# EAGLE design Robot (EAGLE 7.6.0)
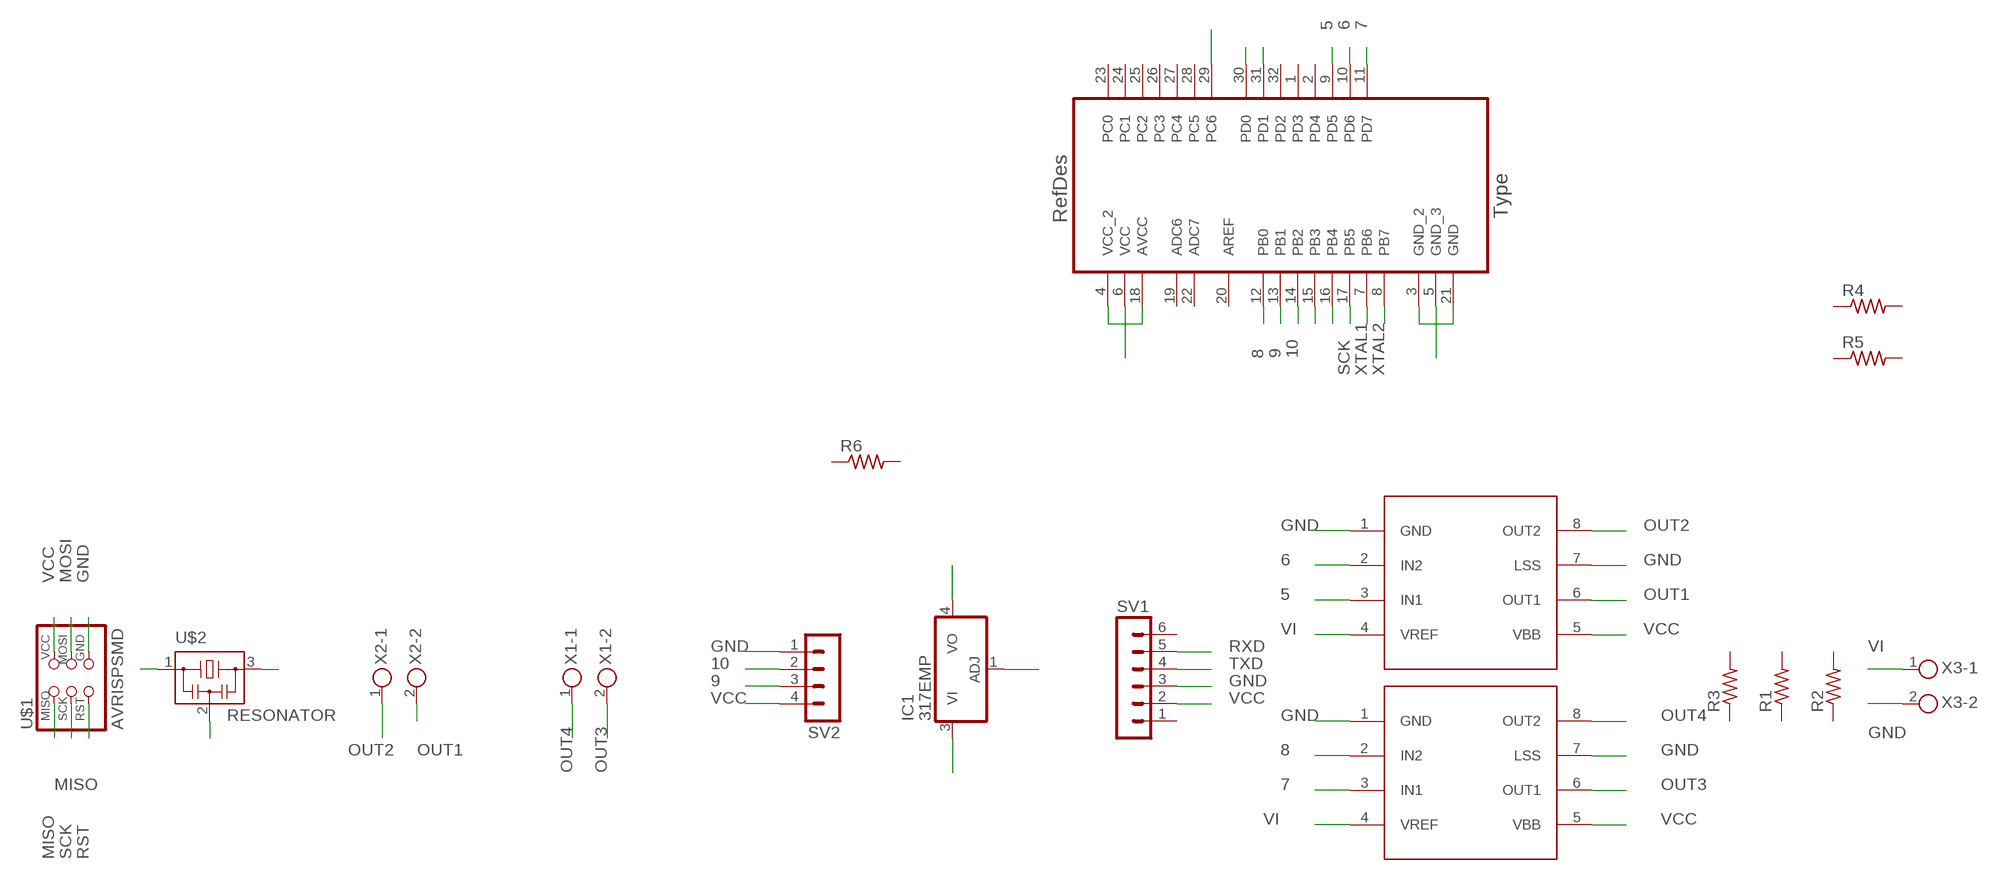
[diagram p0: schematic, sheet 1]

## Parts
IC1  317EMP  [SOT223]
R1  RES-US1206FAB  [R1206FAB]
R2  RES-US1206FAB  [R1206FAB]
R3  RES-US1206FAB  [R1206FAB]
R4  RES-US1206FAB  [R1206FAB]
R5  RES-US1206FAB  [R1206FAB]
R6  RES-US1206FAB  [R1206FAB]
SV1  MA06-1  [MA06-1]
SV2  MA04-1  [MA04-1]
U1  ATMEGA328P-AU  [QFP80P900X900X120-32N]
U$1  AVRISPSMD  [2X03SMD]
U$2  RESONATOR  [EFOBM]
U$3  A4953-H-BRIDGE-MOTOR-DRIVER  [SOIC8]
U$4  A4953-H-BRIDGE-MOTOR-DRIVER  [SOIC8]
X1  AKL59-02  [2POL35]
X2  AKL59-02  [2POL35]
X3  AKL59-02  [2POL35]

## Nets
5: U1.9(PD5) U$3.3(IN1)
6: U1.10(PD6) U$3.2(IN2)
7: U1.11(PD7) U$4.3(IN1)
8: U1.12(PB0) U$4.2(IN2)
9: SV2.3 U1.13(PB1)
10: SV2.2 U1.14(PB2)
GND: IC1.4(VO) SV1.3 SV2.1 U1.3(GND_2) U1.5(GND_3) U1.21(GND) U$1.6(GND) U$2.2 U$3.1(GND) U$3.7(LSS) U$4.1(GND) U$4.7(LSS) X3.2
MISO: U1.16(PB4) U$1.1(MISO)
MOSI: U1.15(PB3) U$1.4(MOSI)
OUT1: U$3.6(OUT1) X2.2
OUT2: U$3.8(OUT2) X2.1
OUT3: U$4.6(OUT1) X1.2
OUT4: U$4.8(OUT2) X1.1
RST: U1.29(PC6) U$1.5(RST)
RXD: SV1.5 U1.31(PD1)
SCK: U1.17(PB5) U$1.3(SCK)
TXD: SV1.4 U1.30(PD0)
VCC: IC1.3(VI) SV1.2 SV2.4 U1.4(VCC_2) U1.6(VCC) U1.18(AVCC) U$1.2(VCC) U$3.5(VBB) U$4.5(VBB)
VI: IC1.1(ADJ) U$3.4(VREF) U$4.4(VREF) X3.1
XTAL1: U1.7(PB6) U$2.3
XTAL2: U1.8(PB7) U$2.1
Unconnected: R1.1 R1.2 R2.1 R2.2 R3.1 R3.2 R4.1 R4.2 R5.1 R5.2 R6.1 R6.2 SV1.1 SV1.6 U1.1(PD3) U1.2(PD4) U1.19(ADC6) U1.20(AREF) U1.22(ADC7) U1.23(PC0) U1.24(PC1) U1.25(PC2) U1.26(PC3) U1.27(PC4) U1.28(PC5) U1.32(PD2)

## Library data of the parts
IC1 = linear:*317: Positive VOLTAGE REGULATOR
R1-R6 = fab:RES-US: Resistor (US Symbol)
SV1 = con-lstb:MA06-1: PIN HEADER; OC_FARNELL: unknown; OC_NEWARK: unknown
SV2 = con-lstb:MA04-1: PIN HEADER; OC_FARNELL: unknown; OC_NEWARK: unknown
U1 = Atmel-ATMEGA328P-AU:ATMEGA328P-AU; DESCRIPTION: 8-bit Microcontroller with In-System Programmable Flash; MPN: ATMEGA328P-AU; OC_FARNELL: 1715486; OC_NEWARK: 14R4631; PACKAGE: TQFP-32; SUPPLIER: Atmel
U$1 = fab:AVRISP
U$2 = fab:RESONATOR
U$3 U$4 = fab:A4953-H-BRIDGE-MOTOR-DRIVER
X1-X3 = con-ria-59:AKL59-02: RIA Anschlussklemme Typ 59, Raster 3,5 mm, Polzahl 2

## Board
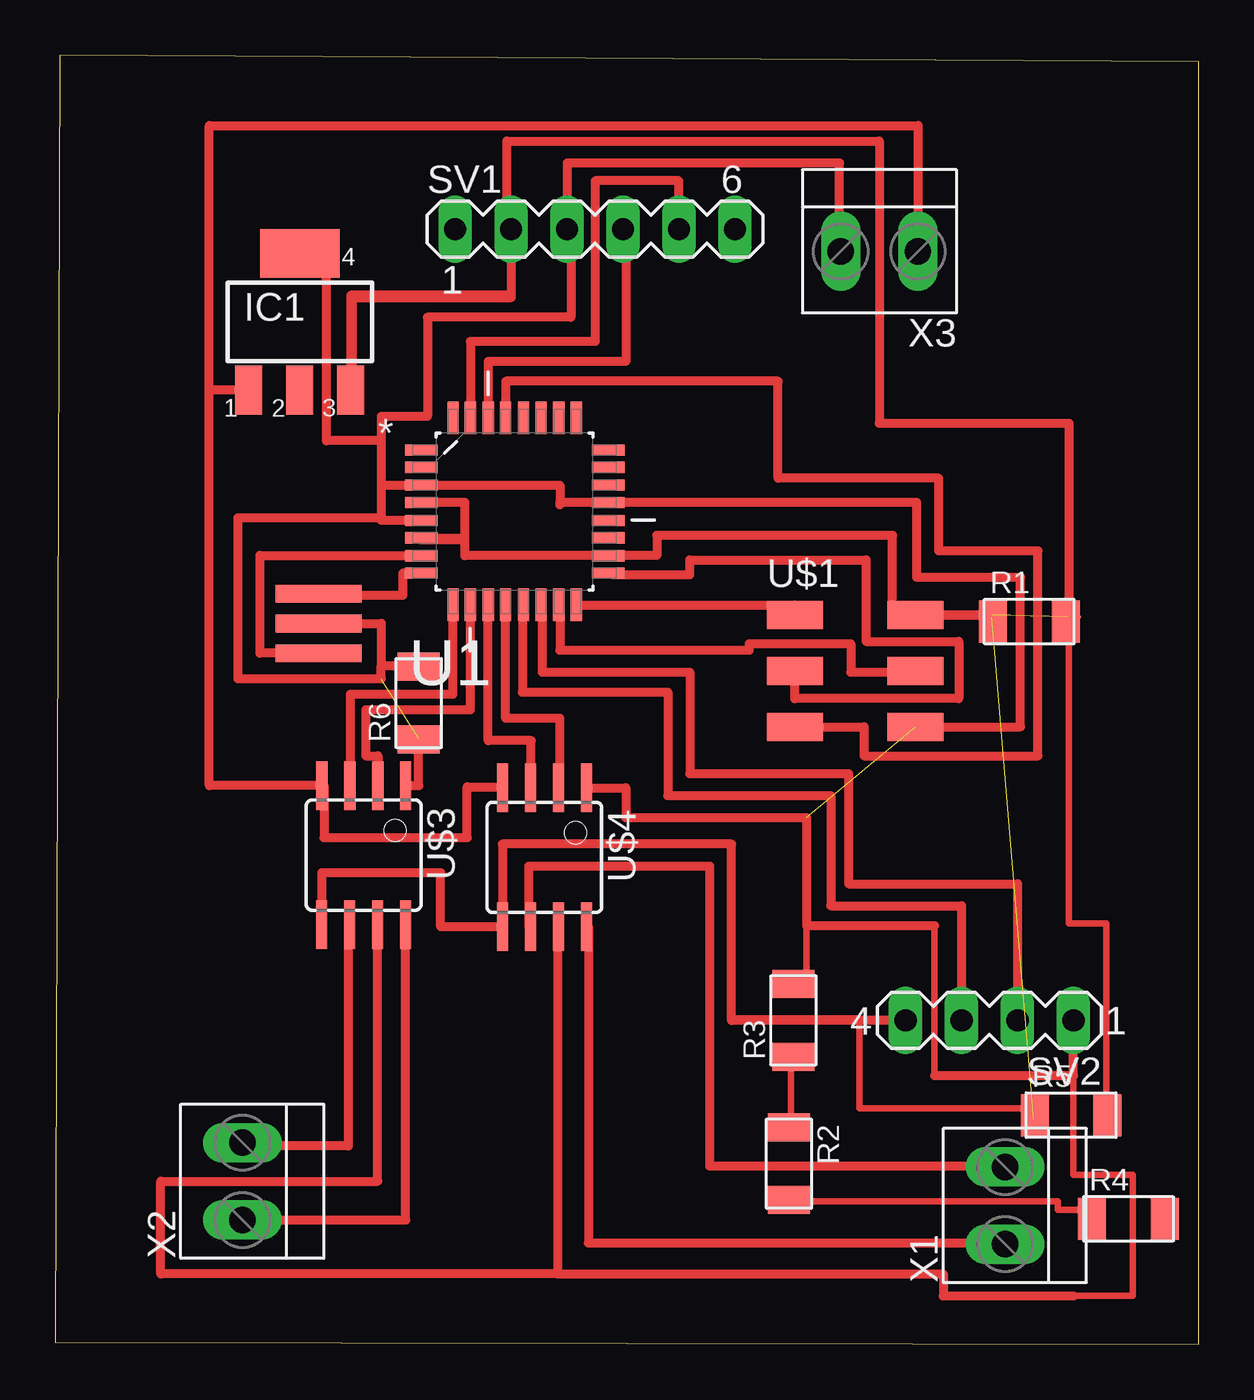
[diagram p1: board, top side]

Size 51.9 x 58.5 mm. Coordinates in mm from the lower left corner, seen from the top.
Outline: 0,0.1 51.9,0 51.9,58.2 0.2,58.5 0,0.1
Copper layers (1*16): Top 0.035mm / dielectric 1.5mm / Bottom 0.035mm
Design rules "default": minimum track width 10mil, minimum drill 24mil, track to track 8mil, track to pad 8mil, pad to pad 8mil, via to via 8mil, smd to smd 8mil, copper to edge 40mil, drill to drill 8mil, minimum pad ring 10mil, minimum via ring 8mil, stop-mask expansion 4mil, vias tented up to drill 0mil, thermal gap 10mil

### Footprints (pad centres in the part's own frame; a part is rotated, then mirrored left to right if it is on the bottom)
SOT223 = smd 1.219 x 2.235: 1 -2.311,-3.099; 2 0,-3.099; 3 2.311,-3.099 | smd 3.6 x 2.2: 4 0,3.099
R1206FAB = smd 1.27 x 1.905: 1 -1.651,0; 2 1.651,0
MA06-1 = drill 1.016 long: 1 -6.35,0; 2 -3.81,0; 3 -1.27,0; 4 1.27,0; 5 3.81,0; 6 6.35,0
MA04-1 = drill 1.016 long: 1 -3.81,0; 2 -1.27,0; 3 1.27,0; 4 3.81,0
QFP80P900X900X120-32N = smd 1.473 x 0.508: 1 -4.242,2.794; 2 -4.242,2.007; 3 -4.242,1.194; 4 -4.242,0.406; 5 -4.242,-0.406; 6 -4.242,-1.194; 7 -4.242,-2.007; 8 -4.242,-2.794; 17 4.242,-2.794; 18 4.242,-2.007; 19 4.242,-1.194; 20 4.242,-0.406; 21 4.242,0.406; 22 4.242,1.194; 23 4.242,2.007; 24 4.242,2.794 | smd 0.508 x 1.473: 9 -2.794,-4.242; 10 -2.007,-4.242; 11 -1.194,-4.242; 12 -0.406,-4.242; 13 0.406,-4.242; 14 1.194,-4.242; 15 2.007,-4.242; 16 2.794,-4.242; 25 2.794,4.242; 26 2.007,4.242; 27 1.194,4.242; 28 0.406,4.242; 29 -0.406,4.242; 30 -1.194,4.242; 31 -2.007,4.242; 32 -2.794,4.242
2X03SMD = smd 2.54 x 1.27: 1 -2.54,2.54; 2 2.92,2.54; 3 -2.54,0; 4 2.92,0; 5 -2.54,-2.54; 6 2.92,-2.54
EFOBM = smd 0.8 x 3.9: 1 -1.35,0; 2 0,0; 3 1.35,0
SOIC8 = smd 0.5 x 2.2: 1 -1.905,-3.154; 2 -0.645,-3.154; 3 0.625,-3.154; 4 1.895,-3.154; 5 1.905,3.154; 6 0.635,3.154; 7 -0.635,3.154; 8 -1.905,3.154
2POL35 = drill 1.2 long: 1 -1.75,0; 2 1.75,0

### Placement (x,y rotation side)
IC1  11.1,46.4 0 top
R1  44.2,32.8 0 top
R2  33.3,8.2 270 top
R3  33.5,14.7 90 top
R4  48.7,5.7 0 top
R5  46.1,10.4 0 top
R6  16.5,29.1 90 top
SV1  24.5,50.6 0 top
SV2  42.4,14.7 180 top
U1  20.85,37.79 0 top
U$1  36.11,30.56 0 top
U$2  11.96,32.71 270 top
U$3  14,22.2 180 top
U$4  22.2,22.1 180 top
X1  43.1,6.3 90 top
X2  8.5,7.4 90 top
X3  37.4,49.6 180 top

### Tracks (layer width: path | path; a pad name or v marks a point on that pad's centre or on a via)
5
  Top 0.406: U$3.3 13.4,25.35 13.4,29.5 18.06,29.5 U1.9
6
  Top 0.406: 14.7,25.35 U$3.2 14.65,26.7 14.1,26.7 14.1,28.8 18.84,28.8 U1.10
7
  Top 0.406: U$4.3 21.6,25.25 21.6,27.4 19.66,27.4 U1.11
8
  Top 0.406: U$4.2 22.9,25.25 22.9,28.4 20.44,28.4 U1.12
9
  Top 0.406: U1.13 21.2,33.55 21.2,29.6 27.8,29.6 27.8,24.9 35.2,24.9 35.2,19.9 41.13,19.9 SV2.3
10
  Top 0.406: U1.14 22.1,33.55 22.1,30.5 28.8,30.5 28.8,25.9 36,25.9 36,20.9 43.67,20.9 SV2.2
GND  (2 unrouted)
  Top 0.305: 39.9,19 39.9,12.2 | 46.21,2.2 48.9,2.2 48.9,7.7 46.21,7.7 46.21,12.2 | 33.4,16.3 34.1,16.3 34.1,19
  Top 0.406: 22.9,38.2 22.9,38.98 U1.3 16.61,39 14.8,39 | 22.9,38.2 U1.21 39.1,38.2 39.1,34.8 43.8,34.8 43.8,28.02 U$1.6 | 22.9,38.2 22.9,38.1 | X3.2 35.6,49.6 35.6,53.6 23.23,53.6 SV1.3 23.4,50.6 23.4,46.6 16.9,46.6 16.9,42.1 14.8,42.1 14.8,41 | U1.5 14.8,37.38 14.8,37.5 | U$2.2 14.8,32.71 14.8,30.8 | 14.8,39 14.8,37.5 | 14.8,37.5 8.3,37.5 8.3,30.2 14.8,30.2 14.8,30.8 | 14.8,41 14.8,39 | 22.8,3.2 4.8,3.2 4.8,7.4 14.63,7.4 U$3.7 | U$4.1 25.9,25.25 25.9,23.9 34.1,23.9 34.1,19 39.9,19 | 39.9,12.2 46.21,12.2 SV2.1 | U$4.7 22.8,18.95 22.8,3.2 | 22.8,3.2 40.3,3.2 40.3,2.2 46.21,2.2 | IC1.4 12.3,49.5 12.3,41 14.8,41 | 14.8,30.8 16.6,30.8 | U$3.1 16.5,25.35 16.5,27.5
MISO
  Top 0.406: U1.16 33.57,33.55 U$1.1
MOSI
  Top 0.406: U1.15 22.9,33.55 22.9,31.5 31.5,31.5 31.5,31.8 36.1,31.8 36.1,30.5 39.03,30.5 U$1.4
N$1
  Top 0.406: 42.7,33.1 39.1,33.1 39.1,33.3
N$2
  Top 0.305: 46.4,33 46,33 46,19.1 47.7,19.1 47.7,10.3
N$3
  Top 0.305: 47,6.1 45.5,6.1 45.5,6.5 33.3,6.5
N$4
  Top 0.406: 10.9,49.3 10.9,49.4
N$5
  Top 0.305: 33.1,9.8 33.4,9.8 33.4,13.3
OUT1
  Top 0.406: U$3.6 13.3,19.05 13.3,9 8.5,9 X2.2
OUT2
  Top 0.406: X2.1 15.91,5.65 U$3.8
OUT3
  Top 0.406: U$4.6 21.5,18.95 21.5,21.7 29.7,21.7 29.7,8.1 43.1,8.1 X1.2
OUT4
  Top 0.406: U$4.8 24.2,18.95 24.2,4.6 43.1,4.6 X1.1
RST
  Top 0.406: U$1.5 36.7,28.02 36.7,26.7 44.6,26.7 44.6,36 40.1,36 40.1,39.3 32.8,39.3 32.8,43.7 20.44,43.7 U1.29
RXD
  Top 0.406: SV1.5 28.3,49.5 28.3,52.8 24.5,52.8 24.5,45.5 18.84,45.5 U1.31
SCK
  Top 0.254: 25.3,34.92 U1.17
  Top 0.406: 25.3,34.92 28.8,34.92 28.8,35.6 36.8,35.6 36.8,31.9 41,31.9 41,29.3 33.57,29.3 U$1.3
TXD
  Top 0.406: SV1.4 25.9,49.5 25.9,44.6 19.66,44.6 U1.30
VCC  (2 unrouted)
  Top 0.305: 30.7,14.8 36.5,14.8 36.5,10.7 44.4,10.7 44.4,10.2
  Top 0.406: U1.4 18.6,38.2 18.6,36.6 U1.6 16.61,36.5 18.6,36.5 18.6,35.78 U1.18 25.09,35.8 27.3,35.8 27.3,36.7 38,36.7 38,33.1 U$1.2 42.5,33.1 42.5,33 | U$3.5 12.09,21.4 17.5,21.4 17.5,18.95 U$4.5 20.3,22.7 30.7,22.7 30.7,14.8 30.7,14.7 SV2.4 | SV1.2 20.7,50.5 | 20.7,50.5 20.7,47.6 | 20.7,47.6 13.41,47.6 IC1.3 13.5,43.3 13.5,47.5 20.7,47.5 20.7,47.6 | 20.7,50.5 20.5,50.5 20.5,54.6 37.4,54.6 37.4,41.8 46,41.8 46,33
VI
  Top 0.406: IC1.1 7,43.3 | 7,43.3 7,55.3 39.15,55.3 X3.1 | U$4.4 20.31,25.3 18.7,25.3 18.7,23 12.2,23 12.2,25.35 U$3.4 7,25.35 7,43.3
XTAL1
  Top 0.406: U$2.3 9.3,31.36 9.3,35.8 16.61,35.8 U1.7
XTAL2
  Top 0.406: U1.8 15.77,35 15.77,33.98 11.96,33.98 U$2.1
